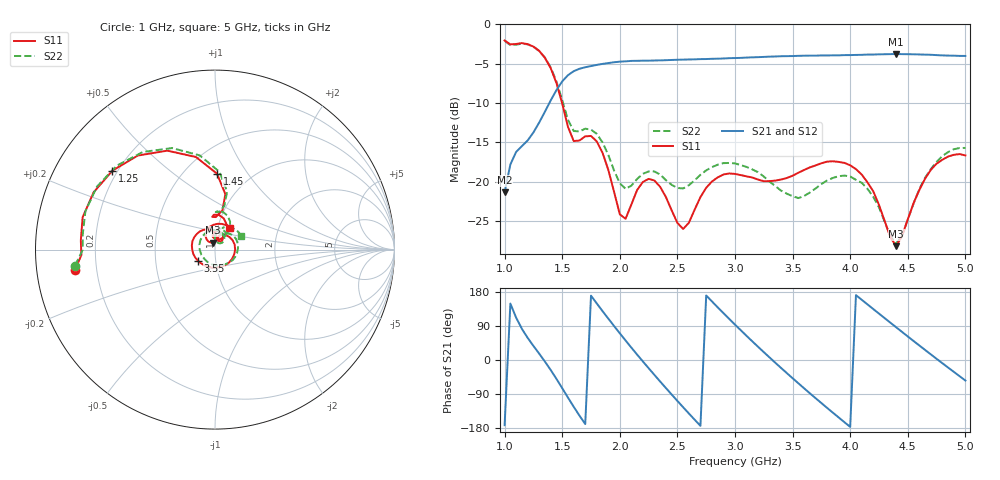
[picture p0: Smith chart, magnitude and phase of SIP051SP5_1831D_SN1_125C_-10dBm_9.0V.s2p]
# GHz  S  dB  R  50
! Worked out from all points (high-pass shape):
!   81 points, 1 GHz to 5 GHz, reference 50 ohm
!   highest |S21| = -3.78 dB at 4.4 GHz (marker M1); lowest = -21.3 dB at 1 GHz (marker M2)
!   |S21| within 3 dB of the highest: 1.53 GHz to end of sweep
!   lowest |S11| = -28.2 dB at 4.4 GHz (marker M3), VSWR 1.08, Z = 48.9 + j3.71 ohm
!   |S11| at or under -10 dB: 1.499 GHz to end of sweep
!   |S22| runs from -27.8 to -2.1 dB; largest |S21 - S12| = 0.0014
!   S11 on the Smith chart (normalised r, x): 1 GHz: 0.12, -0.07; 1.25 GHz: 0.18, +0.33; 1.45 GHz: 0.71, +0.73; 3.55 GHz: 0.82, -0.10; 5 GHz: 1.14, +0.28
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1  -2.06 -171.5  -21.34 -172.1  -21.34 -172.1  -2.11 -173.5
1.25  -2.84 142.4  -13.74 37.2  -13.74 37.3  -2.85 139.5
1.45  -7.46 88.5  -8.36 -49.8  -8.35 -49.7  -7.26 86.7
1.55  -13.03 79.2  -6.47 -99.2  -6.46 -99.2  -12.13 77.9
1.7  -14.23 91.8  -5.46 -169.0  -5.44 -169.0  -13.26 85.4
1.85  -16.32 64.3  -5.04 129.0  -5.03 129.0  -15.00 61.8
2  -24.13 65.9  -4.75 70.5  -4.74 70.6  -20.19 59.6
2.15  -21.06 97.8  -4.64 14.4  -4.65 14.4  -19.65 76.6
2.35  -20.64 62.5  -4.59 -56.6  -4.58 -56.6  -19.08 58.3
2.5  -25.23 55.9  -4.51 -108.0  -4.51 -107.9  -20.79 54.4
2.7  -21.94 72.8  -4.43 -173.8  -4.43 -173.7  -19.11 53.7
2.85  -19.45 41.3  -4.37 138.9  -4.37 138.9  -17.84 35.3
3  -19.00 0.7  -4.29 93.3  -4.28 93.3  -17.67 10.2
3.3  -19.92 -86.8  -4.11 6.7  -4.12 6.7  -19.98 -54.0
3.55  -18.86 -147.6  -4.01 -61.5  -4.01 -61.5  -22.08 -139.6
3.7  -17.93 -180.0  -3.98 -100.9  -3.98 -100.8  -20.85 163.8
4  -17.91 119.8  -3.92 -176.5  -3.92 -176.4  -19.32 84.4
4.15  -20.08 93.2  -3.85 146.7  -3.85 146.7  -20.89 55.7
4.35  -27.09 88.4  -3.79 98.2  -3.80 98.2  -26.95 49.7
4.4  -28.18 104.1  -3.78 86.1  -3.78 86.1  -27.83 63.8
4.7  -18.49 110.9  -3.88 14.8  -3.88 14.8  -18.39 75.7
5  -16.66 56.0  -4.02 -54.2  -4.02 -54.3  -15.71 27.0
